PROGRAM TCPServer
VAR
	
	bSuccess					: BOOL;//函数 F_CreateServerHnd 用于初始化句柄 hServer 内部参数并创建服务器，bSuccess确认是否建立成功
	bEnable						: BOOL;//是否启用
	Step						: INT;
	iCount						: INT;

	//控制器做 TCPIP 的 Server
	sRemoteHost 				: STRING(15) := '169.254.97.15';//控制器IP地址
	nRemotePort 				: UDINT := 2000;//控制器端口号
	fb_ServerConnection			: FB_ServerClientConnection;//建立server 和client连接
	hServer						: T_HSERVER;//TCPIP被创建的服务器
	hSocket						: T_HSOCKET;//TCPIP句柄

	//数据接收
	fb_Receive					: FB_SocketReceive;
	Data_receive				: ARRAY[1..10]OF BYTE;
	bReceive					: BOOL;//接收执行
	
	//数据发送
	fb_Send						: FB_SocketSend;
	nSendDataBuffer	   AT%I*	: ARRAY[1..50]OF BYTE;
	bsend						: BOOL;//发送执行

END_VAR

FBD();
CASE step OF
0:
	bSuccess:=FALSE;
    bEnable:=FALSE;
         step:=step+1;
1:
	bSuccess:=F_CreateServerHnd(
	sSrvNetID:='' ,
	sLocalHost:=sRemoteHost ,
	nLocalPort:=nRemotePort ,
	nMode:=LISTEN_MODE_CLOSEALL OR CONNECT_MODE_ENABLEDBG ,
	bEnable:=TRUE ,
	hServer:=hserver );
         step:=step+1;

2:
        IF bSuccess THEN
 	       bEnable:=TRUE;
	        IF  NOT fb_ServerConnection.bError THEN
		          step:=step+1;
	         ELSE
 		        step:=0;
   	      	END_IF
      	ELSE
	         step:=0;
      	END_IF

3:
		IF fb_ServerConnection.eState=eSOCKET_CONNECTED THEN
				iCount:=iCount+1;
 				step:=step+1;
		END_IF

4:

    fb_Receive(
	sSrvNetId:='' ,
	hSocket:=hSocket ,
	cbLen:=SIZEOF(Data_receive) ,
	pDest:=ADR(Data_receive) ,
	bExecute:=bReceive ,
	tTimeout:=T#1S ,
	bBusy=> ,
	bError=> ,
	nErrId=> ,
	nRecBytes=> );
IF   NOT fb_Receive.bbusy OR NOT fb_Receive.berror THEN
	fb_Send(
	sSrvNetId:='' ,
	hSocket:=hSocket ,
	cbLen:=SIZEOF(nSendDataBuffer) ,
	pSrc:=ADR(nSendDataBuffer) ,
	bExecute:=bsend ,
	tTimeout:=t#6s ,
	bBusy=> ,
	bError=> ,
	nErrId=> );
END_IF
		ELSE
   		 step:=0;

IF bReceive=TRUE THEN
			bReceive:=FALSE;//只接收一次数据
END_IF
IF bsend=TRUE THEN
			bsend:=FALSE;//只发送一次数据
END_IF
END_CASE

ACTION FBD:
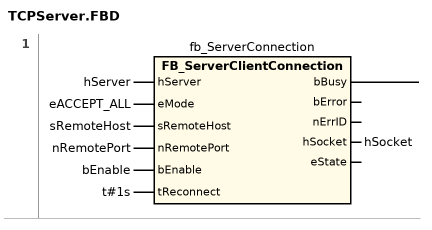
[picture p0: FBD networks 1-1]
// NETWORK 1
fb_ServerConnection(
    hServer := hServer,
    eMode := eACCEPT_ALL,
    sRemoteHost := sRemoteHost,
    nRemotePort := nRemotePort,
    bEnable := bEnable,
    tReconnect := t#1s,
    hSocket => hSocket); // FB_ServerClientConnection
END_ACTION

END_PROGRAM
